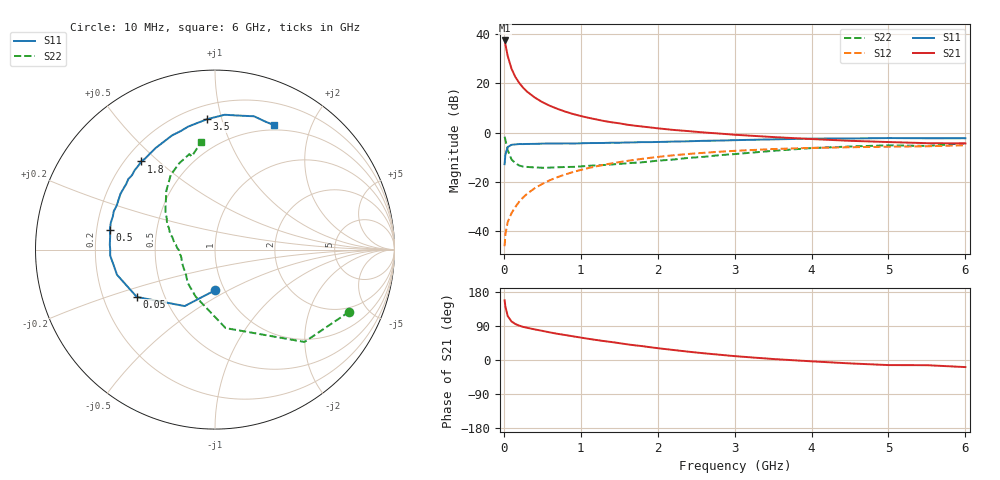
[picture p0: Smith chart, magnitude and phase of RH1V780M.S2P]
! SIEMENS Small Signal Semiconductors
! BFR106
! Si NPN RF Bipolar Junction Transistor in SOT23
! VCE = 1.75 V  IC = 80 mA
! Common Emitter S-Parameters:  August  1996
# GHz  S  MA  R  50
!  f  S11  S21  S12  S22
! GHz  MAG  ANG  MAG  ANG  MAG  ANG  MAG  ANG
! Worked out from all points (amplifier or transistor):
!   36 points, 10 MHz to 6 GHz, reference 50 ohm
!   highest |S21| = 37.5 dB at 10 MHz (marker M1)
!   |S21| within 3 dB of that: start of sweep to 29.33 MHz
!   unconditionally stable (mu >= 1): 148.3 MHz to 3.248 GHz; 4.222 GHz to end of sweep
!   at 250 MHz: K = 1.08, MAG = 20.7 dB, |S12| = -26.4 dB
!   at 1.4 GHz: K = 1.08, MAG = 6.7 dB, |S12| = -12.5 dB
!   at 6 GHz: K = 1.02, MAG = -0.5 dB, |S12| = -5.2 dB
!   S11 on the Smith chart (normalised r, x): 10 MHz: 0.90, -0.43; 50 MHz: 0.35, -0.25; 500 MHz: 0.26, +0.09; 1.8 GHz: 0.26, +0.44; 3.5 GHz: 0.29, +0.90; 6 GHz: 0.44, +1.49
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0.01  0.2278 -90.5  74.68 157.7  0.0049 74.2  0.8243 -24.8
0.02  0.357 -118.2  62.77 141.1  0.0085 65.0  0.7165 -45.9
0.05  0.5093 -148.8  36.14 116.0  0.0151 59.4  0.4412 -82.3
0.1  0.5638 -165.6  19.85 101.6  0.023 64.1  0.2834 -112.3
0.15  0.5751 -173.1  13.48 94.9  0.0308 67.7  0.2399 -129.3
0.2  0.5847 -176.6  10.23 90.7  0.0394 70.2  0.2135 -139.3
0.25  0.5837 179.9  8.181 87.4  0.0478 71.7  0.2038 -148.1
0.3  0.5867 177.4  6.85 85.1  0.0565 72.5  0.2005 -152.8
0.4  0.5891 172.5  5.182 80.8  0.0736 72.7  0.1953 -161.0
0.5  0.5962 169.3  4.164 76.9  0.0905 72.1  0.1929 -166.5
0.6  0.5996 165.5  3.494 72.8  0.1078 71.2  0.1936 -169.8
0.7  0.5983 162.1  3.024 69.0  0.1245 69.8  0.1972 -172.8
0.9  0.6 155.9  2.386 62.5  0.1578 66.9  0.2006 -178.9
1.1  0.6117 149.3  1.997 55.9  0.1901 63.6  0.211 177.5
1.4  0.6227 140.9  1.621 47.4  0.2362 58.3  0.2245 171.4
1.8  0.6404 129.9  1.327 36.6  0.2927 51.3  0.2487 163.5
2.2  0.6555 120.3  1.134 26.5  0.3448 44.2  0.2826 155.2
2.8  0.687 106.3  0.956 14.0  0.4071 33.9  0.3467 142.7
3.5  0.7278 93.5  0.811 2.6  0.4627 22.7  0.4254 129.6
4.5  0.759 79.5  0.68 -9.0  0.5032 8.6  0.5208 112.4
5.5  0.7664 68.5  0.609 -13.7  0.5266 0.2  0.5355 103.9
6  0.7673 64.5  0.602 -18.7  0.552 -6.4  0.6068 97.2
